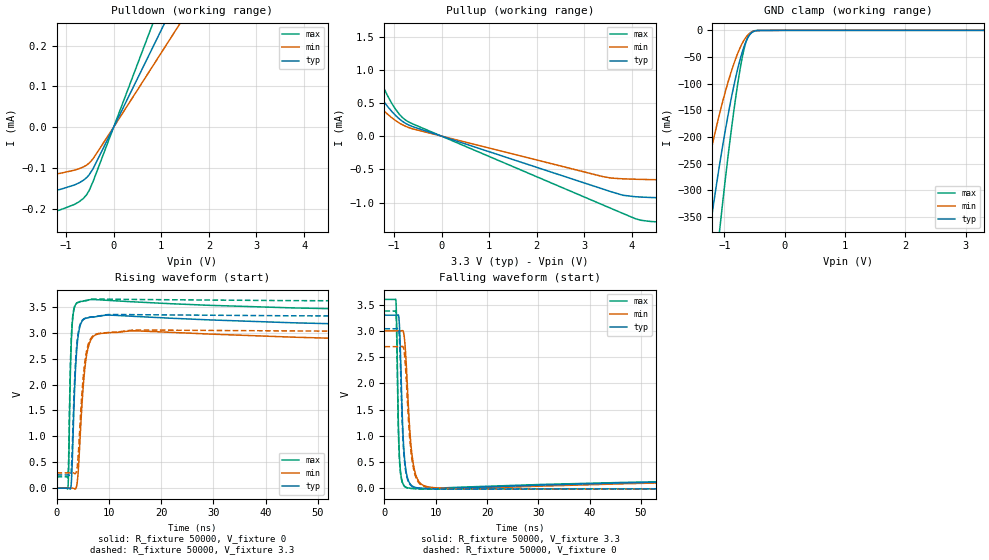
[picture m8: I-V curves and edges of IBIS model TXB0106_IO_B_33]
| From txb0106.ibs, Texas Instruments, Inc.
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[Model]   TXB0106_IO_B_33
Model_type  I/O
Vinl=1.05
Vinh=2.34
Enable   Active-High
Vref =   0
Rref =   1e6
Cref =   15p
Vmeas =   1.65
| variable   typ   min   max
C_comp   13.90pF   11.82pF   15.62pF
| C_pullup   13.81pF   11.79pF   15.76pF
| C_pulldown   21.52pF   11.45pF   39.52pF
| C_tri-state   13.90pF   11.82pF   15.62pF
[Temperature Range]   40   100   -40
| Ambient temperature   25   85   -40
[Voltage range]   3.3   3   3.6
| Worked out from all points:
|   slope of the pulldown table from 0 to 0.495 V, typ, clamps not added: 4.2 kohm
|   slope of the pullup table from 0 to 0.495 V, typ, clamps not added: 4.25 kohm
|   GND clamp passes 1 mA (typ) near -0.48 V on its own axis
|   rising waveform, R_fixture 50000, V_fixture 0: 20-80 % time 669ps typ, 998ps min, 409ps max; typ from 0 V to 3.05 V
|   falling waveform, R_fixture 50000, V_fixture 3.3: 20-80 % time 628ps typ, 980ps min, 386ps max; typ from 3.3 V to 0.246 V
|   rising waveform, R_fixture 50000, V_fixture 3.3: 20-80 % time 770ps typ, 1.18ns min, 459ps max; typ from 0.256 V to 3.3 V
|   falling waveform, R_fixture 50000, V_fixture 0: 20-80 % time 738ps typ, 1.18ns min, 434ps max; typ from 3.04 V to 0 V
[GND Clamp]
| TXB0104_IO_B_33
|   Voltage   I(typ)   I(min)   I(max)
-5.5V     -5.138A    -3.901A    -6.439A
-1.49V    -586.4mA   -378.2mA   -853.1mA
-1.44V    -541.6mA   -347.7mA   -791.1mA
-1.245V   -376.5mA   -237.5mA   -558.3mA
-1.22V    -356.6mA   -224.4mA   -529.6mA
-1.085V   -255.2mA   -158.5mA   -381mA
-1.065V   -241mA     -149.4mA   -360mA
-890mV    -129.5mA   -78.64mA   -190.6mA
-740mV    -54.71mA   -32.62mA   -72.62mA
-640mV    -20.32mA   -12.58mA   -21.08mA
-545mV    -4.204mA   -3.114mA   -2.676mA
3.3V      891.3pA    4.328nA    103.8pA
[Pulldown]
| TXB0104_IO_B_33
|   Voltage   I(typ)   I(min)   I(max)
-5.5V     -213uA     -161uA     -279uA
-3.115V   -186uA     -140uA     -247uA
-2.585V   -179uA     -134uA     -239uA
-1.64V    -164.4uA   -122.2uA   -219uA
-1.125V   -152.7uA   -113.2uA   -202.8uA
-825mV    -141.8uA   -105.5uA   -189.5uA
-635mV    -130.1uA   -97.48uA   -174.6uA
-570mV    -123.9uA   -93.19uA   -165.9uA
-515mV    -116.8uA   -88.24uA   -155.4uA
-430mV    -101.3uA   -77.17uA   -132.5uA
0V        0A         0A         0A
11V       2.618mA    2.005mA    3.396mA
[Pullup]
| TXB0104_IO_B_33
|   Voltage   I(typ)   I(min)   I(max)
-5.5V     3.568mA    1.757mA    6.305mA
-2.22V    2.391mA    1.681mA    3.337mA
-2.01V    1.736mA    1.251mA    2.479mA
-1.95V    1.592mA    1.149mA    2.297mA
-1.705V   1.139mA    818.9uA    1.675mA
-1.225V   535uA      392.4uA    743.4uA
-965mV    311.4uA    235.2uA    403.8uA
-765mV    196.9uA    152uA      247.2uA
3.39V     -796.7uA   -609.3uA   -1.036mA
4.185V    -916.9uA   -650.6uA   -1.266mA
5.975V    -947uA     -669uA     -1.327mA
11V       -978uA     -690uA     -1.373mA
[Ramp]
| TXB0104_IO_B_33
| variable   typ   min   max
dV/dt_r   2.01/8.09E-10   1.83/1.24E-09   2.20/4.84E-10
dV/dt_f   1.99/7.51E-10   1.81/1.20E-09   2.17/4.47E-10
R_load = 50000
[Rising Waveform]
| TXB0104_IO_B_33
R_fixture =   50000
C_fixture =   0
L_fixture =   0
V_fixture =   0
V_fixture_min = 0
V_fixture_max = 0
|   Time   V(typ)   V(min)   V(max)
0s        144.2nV    1.32uV     44.14nV
2.175ns   144.8uV    4.908uV    918.9uV
2.32ns    1.042mV    3.307uV    383.8mV
2.655ns   -14.3mV    -126.3uV   2.252V
2.88ns    189.1mV    418.5uV    2.944V
3.46ns    1.908V     -12.26mV   3.498V
3.84ns    2.635V     35.98mV    3.567V
5.29ns    3.264V     2.181V     3.614V
6.43ns    3.299V     2.832V     3.638V
220ns     3.046V     2.715V     3.38V
[Falling Waveform]
| TXB0104_IO_B_33
R_fixture =   50000
C_fixture =   0
L_fixture =   0
V_fixture =   3.3
V_fixture_min = 3
V_fixture_max = 3.6
|   Time   V(typ)   V(min)   V(max)
0s        3.3V       3V         3.6V
2.225ns   3.3V       3V         3.585V
2.375ns   3.299V     3V         3.157V
2.78ns    3.279V     3V         980.3mV
3.135ns   2.527V     2.999V     318.4mV
3.8ns     720mV      2.93V      56.89mV
5.025ns   84.53mV    992.8mV    3.342mV
6.67ns    9.417mV    136.8mV    -4.612mV
11.8ns    -257.3uV   2.17mV     12.55mV
220ns     246.2mV    273mV      215.8mV
[Rising Waveform]
| TXB0104_IO_B_33
R_fixture =   50000
C_fixture =   0
L_fixture =   0
V_fixture =   3.3
V_fixture_min = 3
V_fixture_max = 3.6
|   Time   V(typ)   V(min)   V(max)
0s        255.5mV    296.2mV    218.9mV
2.18ns    255.7mV    296.2mV    224mV
2.31ns    256.7mV    296.2mV    561.7mV
2.74ns    272.3mV    296.1mV    2.685V
3.265ns   1.575V     292.8mV    3.434V
3.705ns   2.547V     291mV      3.558V
4.23ns    3.047V     757.1mV    3.59V
5.26ns    3.269V     2.299V     3.616V
6.49ns    3.304V     2.876V     3.645V
220ns     3.301V     3.002V     3.6V
[Falling Waveform]
| TXB0104_IO_B_33
R_fixture =   50000
C_fixture =   0
L_fixture =   0
V_fixture =   0
V_fixture_min = 0
V_fixture_max = 0
|   Time   V(typ)   V(min)   V(max)
0s        3.041V     2.7V       3.379V
2.225ns   3.041V     2.7V       3.365V
2.37ns    3.041V     2.7V       2.964V
2.775ns   3.024V     2.7V       891.2mV
3.13ns    2.298V     2.699V     291.7mV
3.775ns   669.6mV    2.646V     54.42mV
4.995ns   74.77mV    875.5mV    2.071mV
6.61ns    6.517mV    119.5mV    -6.845mV
11.47ns   -12.17mV   -84uV      -10.55mV
220ns     -493.7uV   -1.136mV   -175.5uV
